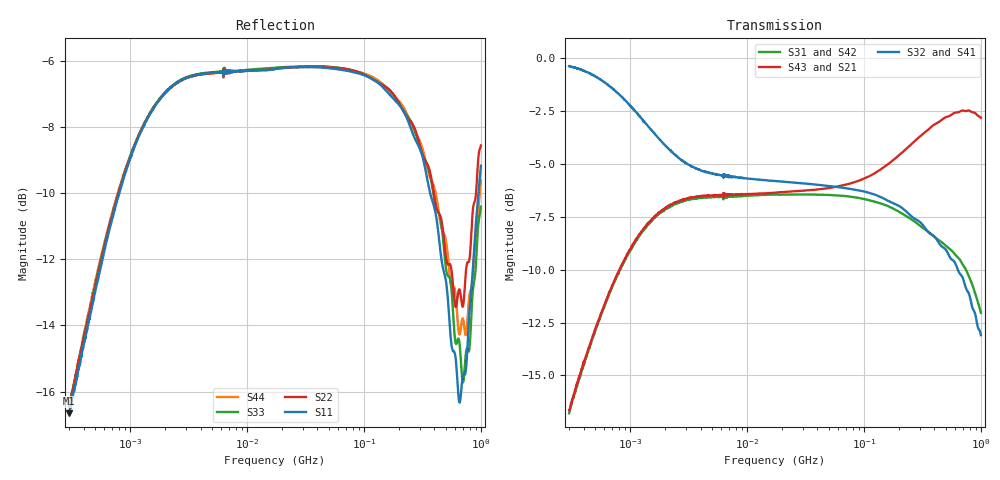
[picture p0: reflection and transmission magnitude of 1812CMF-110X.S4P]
!s-Parameter Generated by FASTRON Sdn. Bhd.
!FASTRON P/N : 1812CMF-110X
!Keysight Technologies: E5071C_MY46733604_B.14.02
!Date: Mon Mar 09 13:24:16 2026
!Version  :Rev00  Mon Mar 09 13:24:16 2026
!Data & Calibration Information:
!Freq	S11:SOLT4(ON)	S12:SOLT4(ON)	S13:SOLT4(ON)	S14:SOLT4(ON)
!	S21:SOLT4(ON)	S22:SOLT4(ON)	S23:SOLT4(ON)	S24:SOLT4(ON)
!	S31:SOLT4(ON)	S32:SOLT4(ON)	S33:SOLT4(ON)	S34:SOLT4(ON)
!	S41:SOLT4(ON)	S42:SOLT4(ON)	S43:SOLT4(ON)	S44:SOLT4(ON)
!PortZ  Port1:50+j0  Port2:50+j0  Port3:50+j0  Port4:50+j0
!When reading reference impedance value at option line is always used.
! Remarks : This data is being provided solely for informational purposes.
# Hz S dB R 50
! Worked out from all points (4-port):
!   1601 points, 300 kHz to 1 GHz, reference 50 ohm
!   strongest paths, dB at 300 kHz, 2.303 MHz, 17.55 MHz, 132.8 MHz, 1 GHz:
!     S32: -0.4, -4.5, -5.8, -6.5, -13.1
!     S41: -0.3, -4.5, -5.8, -6.5, -13.1
!     S43: -16.6, -6.9, -6.4, -5.3, -2.8
!     S21: -16.7, -6.9, -6.4, -5.3, -3.0
!     S31: -16.8, -6.9, -6.4, -6.8, -12.0
!     S42: -16.8, -7.0, -6.5, -6.8, -12.6
!   lowest |S11| = -16.7 dB at 300 kHz (marker M1), VSWR 1.34, Z = 55.5 + j14.6 ohm
!   |S11| at or under -10 dB: start of sweep to 806.5 kHz; 367.7 MHz to 955.2 MHz (587.5 MHz wide, 88.8 % of centre)
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300000  -16.66 61.4  -16.70 72.0  -16.75 -108.5  -0.45 -8.5
        -16.69 71.7  -16.46 63.2  -0.39 -8.9  -16.90 -109.2
        -16.79 -108.5  -0.38 -8.8  -16.37 63.5  -16.84 71.6
        -0.33 -9.1  -16.79 -108.5  -16.65 70.9  -16.39 64.9
1664702  -7.31 28.4  -7.43 29.5  -7.44 -151.1  -3.65 -19.0
         -7.45 29.6  -7.31 28.4  -3.64 -19.0  -7.48 -150.9
         -7.47 -151.0  -3.66 -19.0  -7.29 28.4  -7.44 29.6
         -3.66 -18.9  -7.49 -150.9  -7.40 29.7  -7.32 28.3
8845367  -6.33 4.3  -6.46 6.7  -6.49 -176.2  -5.65 -7.5
         -6.48 6.7  -6.33 4.4  -5.65 -7.5  -6.51 -176.1
         -6.52 -176.1  -5.67 -7.5  -6.31 4.3  -6.47 6.6
         -5.68 -7.4  -6.53 -175.8  -6.44 6.6  -6.32 4.5
6.034632e7  -6.27 -8.8  -6.09 6.0  -6.47 168.2  -6.08 -13.1
            -6.10 6.0  -6.22 -8.4  -6.08 -13.8  -6.52 169.2
            -6.49 168.1  -6.10 -13.8  -6.22 -9.3  -6.09 6.1
            -6.07 -13.1  -6.51 169.0  -6.06 6.1  -6.22 -7.9
3.040119e8  -8.71 -38.0  -3.64 5.9  -7.90 123.6  -7.76 -51.8
            -3.66 5.9  -8.63 -35.3  -7.74 -54.0  -7.88 127.7
            -7.94 123.7  -7.77 -54.0  -8.68 -39.9  -3.69 6.2
            -7.75 -51.7  -7.87 127.7  -3.68 6.1  -8.48 -34.1
6.570262e8  -16.33 -4.7  -2.49 -11.3  -9.49 73.5  -9.78 -101.2
            -2.51 -11.2  -12.91 -9.8  -10.16 -103.9  -9.73 78.8
            -9.51 73.5  -10.17 -104.1  -14.55 -19.6  -2.54 -9.5
            -9.81 -101.1  -9.74 78.9  -2.53 -9.6  -14.27 -16.0
1e9  -9.17 43.8  -2.96 -27.7  -12.04 31.3  -13.05 -145.7
     -2.97 -27.6  -8.56 28.8  -13.10 -151.1  -12.59 38.9
     -12.03 31.3  -13.09 -151.3  -10.41 36.2  -2.83 -24.9
     -13.09 -146.1  -12.60 38.9  -2.82 -24.6  -9.62 31.8
